(* Logix 5000 AddOnInstructionDefinition export B512_HtoD; software revision 30.00 *)

ADD_ON_INSTRUCTION D_SHR   (* revision 1.0, vendor Ken Fischer, NSWCPD, C512 *)
// DINT bit shift right of the 32-bit argument Inp_A by Inp_B bits with paddding by zeros on the right
// Revision note:
// Rev1.0: TBD - Initial Release
VAR_IN_OUT
   Inp_A : DINT; {required}   // 64-bit Integer to be right circular rotated
END_VAR
VAR_INPUT
   Inp_B : INT; {required}   // Number of bits to shift
END_VAR
VAR_IN_OUT
   Out : DINT; {required}   // Result
END_VAR
VAR
   BSR_Cntrl : CONTROL := (LEN := 32);
   ONS : BOOL;
   Source_Bit : BOOL;
   Wrk_InpA : DINT[2];
END_VAR

ROUTINE Logic   (* ladder *)
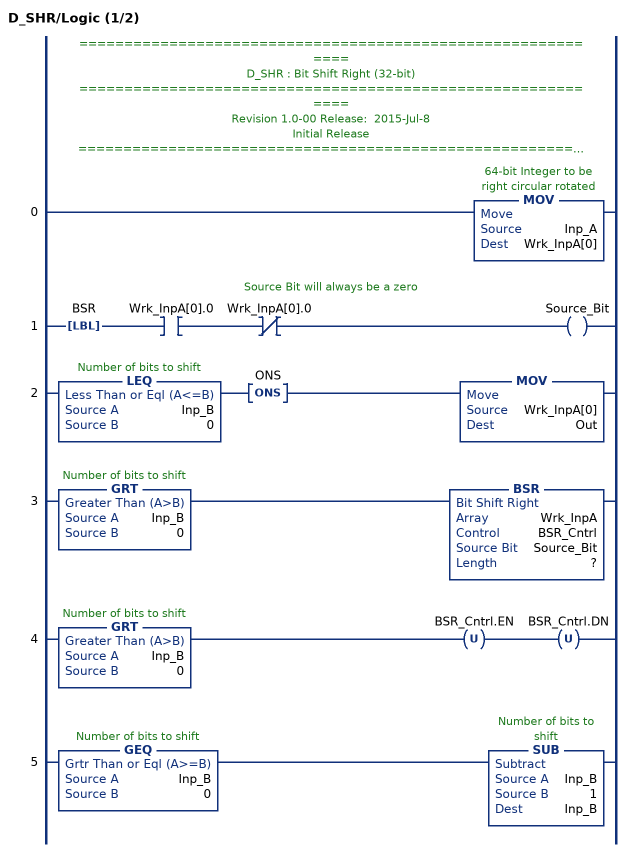
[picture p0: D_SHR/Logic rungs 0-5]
   // ============================================================
   // D_SHR : Bit Shift Right (32-bit)
   // ============================================================
   // Revision 1.0-00 Release:  2015-Jul-8
   // Initial Release
   // ============================================================
   // Performs a right bit shift of the 32-bit argument Inp_A by the
   // number of bits defined in the 16-bit argument Inp_B, with padding by zeros.
   0: MOV(Inp_A,Wrk_InpA[0]);
   // Source Bit will always be a zero
   1: LBL(BSR)XIC(Wrk_InpA[0].0)XIO(Wrk_InpA[0].0)OTE(Source_Bit);
   2: LEQ(Inp_B,0)ONS(ONS)MOV(Wrk_InpA[0],Out);
   3: GRT(Inp_B,0)BSR(Wrk_InpA,BSR_Cntrl,Source_Bit,?);
   4: GRT(Inp_B,0)OTU(BSR_Cntrl.EN)OTU(BSR_Cntrl.DN);
   5: GEQ(Inp_B,0)SUB(Inp_B,1,Inp_B);
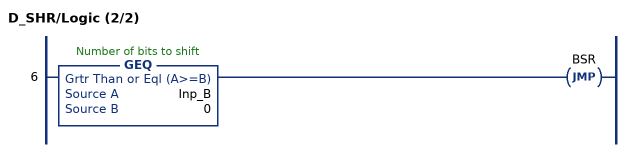
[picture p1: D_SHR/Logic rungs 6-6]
   6: GEQ(Inp_B,0)JMP(BSR);
END_ROUTINE
END_ADD_ON_INSTRUCTION

ADD_ON_INSTRUCTION D_SHL   (* revision 1.0, vendor Ken Fischer, NSWCPD, C512 *)
// DINT bit shift left of the 32-bit argument Inp_A by Inp_B bits with paddding by zeros on the right
// Revision note:
// Rev1.0: TBD - Initial Release
VAR_IN_OUT
   Inp_A : DINT; {required}   // 64-bit Integer to be right circular rotated
END_VAR
VAR_INPUT
   Inp_B : INT; {required}   // Number of bits to shift
END_VAR
VAR_IN_OUT
   Out : DINT; {required}   // Result
END_VAR
VAR
   Wrk_InpA : DINT[2];
   Source_Bit : BOOL;
   ONS : BOOL;
   BSL_Cntrl : CONTROL := (LEN := 32);
END_VAR

ROUTINE Logic   (* ladder *)
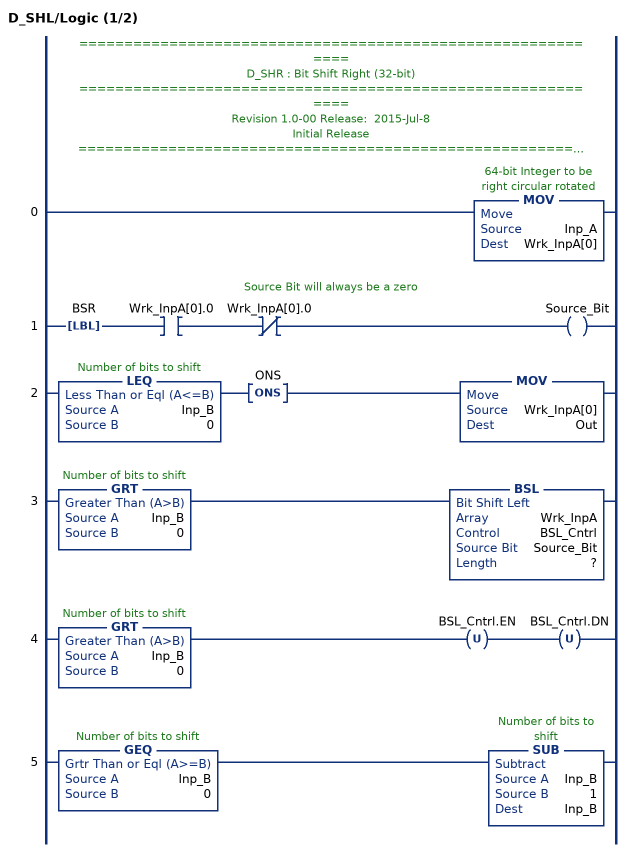
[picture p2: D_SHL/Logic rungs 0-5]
   // ============================================================
   // D_SHR : Bit Shift Right (32-bit)
   // ============================================================
   // Revision 1.0-00 Release:  2015-Jul-8
   // Initial Release
   // ============================================================
   // Performs a left bit shift of the 32-bit argument Inp_A by the
   // number of bits defined in the 16-bit argument Inp_B, with padding by zeros.
   0: MOV(Inp_A,Wrk_InpA[0]);
   // Source Bit will always be a zero
   1: LBL(BSR)XIC(Wrk_InpA[0].0)XIO(Wrk_InpA[0].0)OTE(Source_Bit);
   2: LEQ(Inp_B,0)ONS(ONS)MOV(Wrk_InpA[0],Out);
   3: GRT(Inp_B,0)BSL(Wrk_InpA,BSL_Cntrl,Source_Bit,?);
   4: GRT(Inp_B,0)OTU(BSL_Cntrl.EN)OTU(BSL_Cntrl.DN);
   5: GEQ(Inp_B,0)SUB(Inp_B,1,Inp_B);
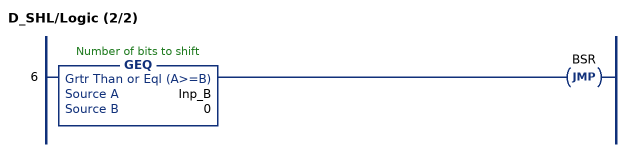
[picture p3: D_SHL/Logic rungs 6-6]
   6: GEQ(Inp_B,0)JMP(BSR);
END_ROUTINE
END_ADD_ON_INSTRUCTION

ADD_ON_INSTRUCTION B512_HtoD   (* revision 1.0 20170916, vendor Kenneth A. Fischer *)
// Takes a 512-bit hash value stored as 8 64-bit pieces and converts it to a 512-bit value stored as 42 12-bit pieces and 1 8-bit piece as the MSB
// Revision note:
// Rev1.0: 20170916 - Initial Release
VAR_IN_OUT
   Inp_H : LINT[8]; {required}
   Out_D : DINT[43]; {required}
END_VAR
VAR
   i : INT := 41;
   j : INT := 62;
   Wrk_InpL : DINT[16];
   D_SHR : D_SHR;
   TEMP1 : DINT;
   D_SHL : D_SHL;
   TEMP2 : DINT;
   EE : DINT[64];
END_VAR

ROUTINE Logic   (* ladder *)
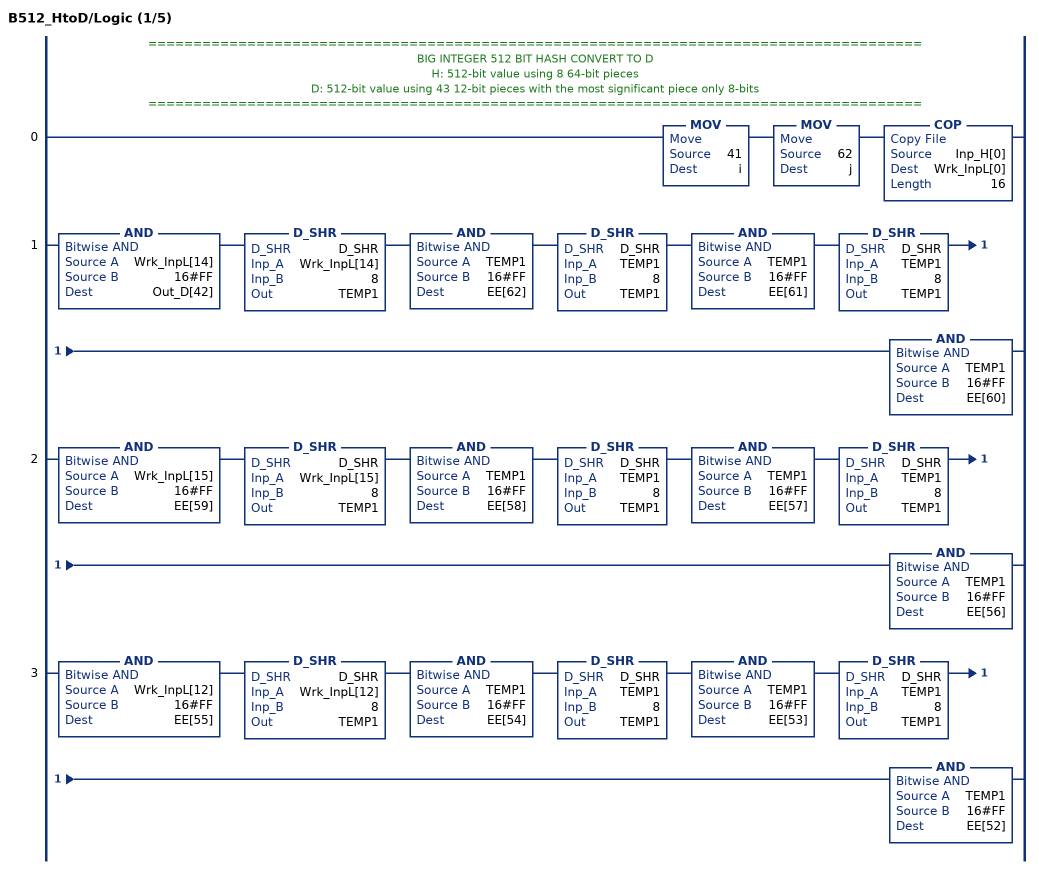
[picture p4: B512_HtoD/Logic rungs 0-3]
   // ======================================================================================
   // BIG INTEGER 512 BIT HASH CONVERT TO D
   // H: 512-bit value using 8 64-bit pieces
   // D: 512-bit value using 43 12-bit pieces with the most significant piece only 8-bits
   // ======================================================================================
   0: MOV(41,i)MOV(62,j)COP(Inp_H[0],Wrk_InpL[0],16);
   1: AND(Wrk_InpL[14],16#FF,Out_D[42])D_SHR(D_SHR,Wrk_InpL[14],8,TEMP1)AND(TEMP1,16#FF,EE[62])D_SHR(D_SHR,TEMP1,8,TEMP1)AND(TEMP1,16#FF,EE[61])D_SHR(D_SHR,TEMP1,8,TEMP1)AND(TEMP1,16#FF,EE[60]);
   2: AND(Wrk_InpL[15],16#FF,EE[59])D_SHR(D_SHR,Wrk_InpL[15],8,TEMP1)AND(TEMP1,16#FF,EE[58])D_SHR(D_SHR,TEMP1,8,TEMP1)AND(TEMP1,16#FF,EE[57])D_SHR(D_SHR,TEMP1,8,TEMP1)AND(TEMP1,16#FF,EE[56]);
   3: AND(Wrk_InpL[12],16#FF,EE[55])D_SHR(D_SHR,Wrk_InpL[12],8,TEMP1)AND(TEMP1,16#FF,EE[54])D_SHR(D_SHR,TEMP1,8,TEMP1)AND(TEMP1,16#FF,EE[53])D_SHR(D_SHR,TEMP1,8,TEMP1)AND(TEMP1,16#FF,EE[52]);
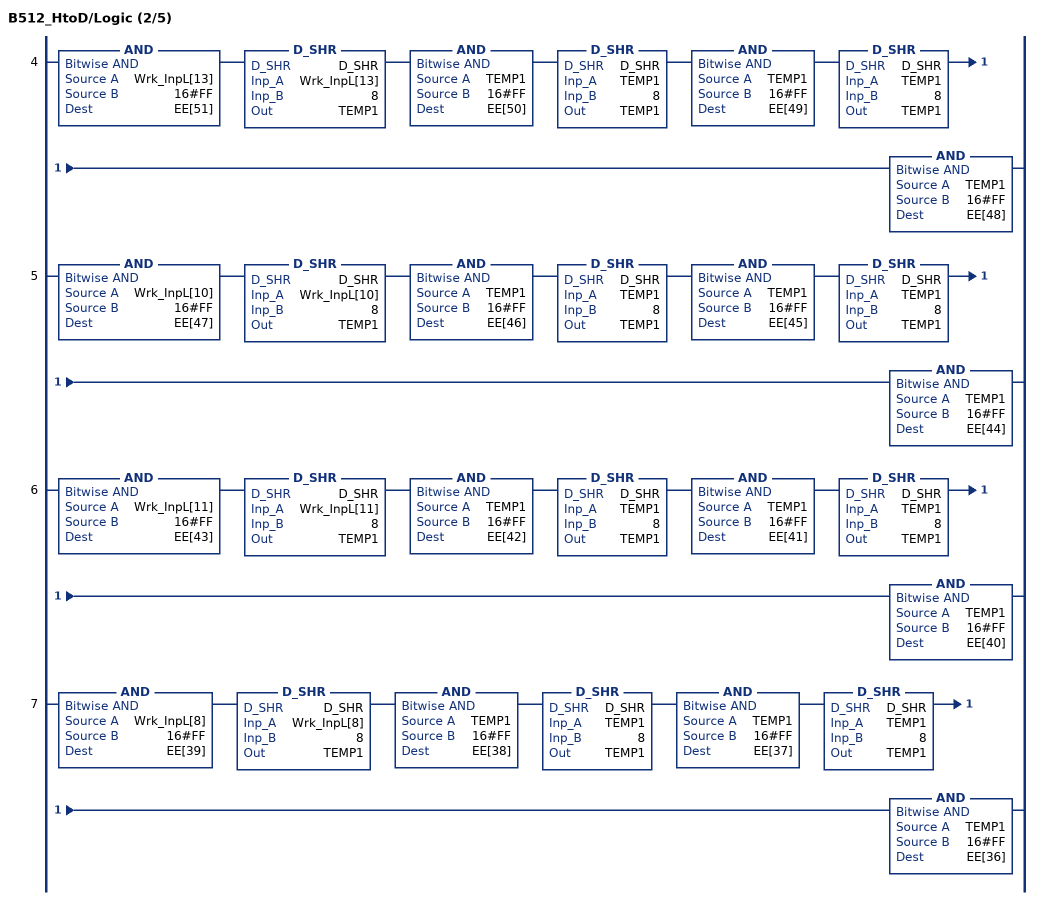
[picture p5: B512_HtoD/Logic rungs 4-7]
   4: AND(Wrk_InpL[13],16#FF,EE[51])D_SHR(D_SHR,Wrk_InpL[13],8,TEMP1)AND(TEMP1,16#FF,EE[50])D_SHR(D_SHR,TEMP1,8,TEMP1)AND(TEMP1,16#FF,EE[49])D_SHR(D_SHR,TEMP1,8,TEMP1)AND(TEMP1,16#FF,EE[48]);
   5: AND(Wrk_InpL[10],16#FF,EE[47])D_SHR(D_SHR,Wrk_InpL[10],8,TEMP1)AND(TEMP1,16#FF,EE[46])D_SHR(D_SHR,TEMP1,8,TEMP1)AND(TEMP1,16#FF,EE[45])D_SHR(D_SHR,TEMP1,8,TEMP1)AND(TEMP1,16#FF,EE[44]);
   6: AND(Wrk_InpL[11],16#FF,EE[43])D_SHR(D_SHR,Wrk_InpL[11],8,TEMP1)AND(TEMP1,16#FF,EE[42])D_SHR(D_SHR,TEMP1,8,TEMP1)AND(TEMP1,16#FF,EE[41])D_SHR(D_SHR,TEMP1,8,TEMP1)AND(TEMP1,16#FF,EE[40]);
   7: AND(Wrk_InpL[8],16#FF,EE[39])D_SHR(D_SHR,Wrk_InpL[8],8,TEMP1)AND(TEMP1,16#FF,EE[38])D_SHR(D_SHR,TEMP1,8,TEMP1)AND(TEMP1,16#FF,EE[37])D_SHR(D_SHR,TEMP1,8,TEMP1)AND(TEMP1,16#FF,EE[36]);
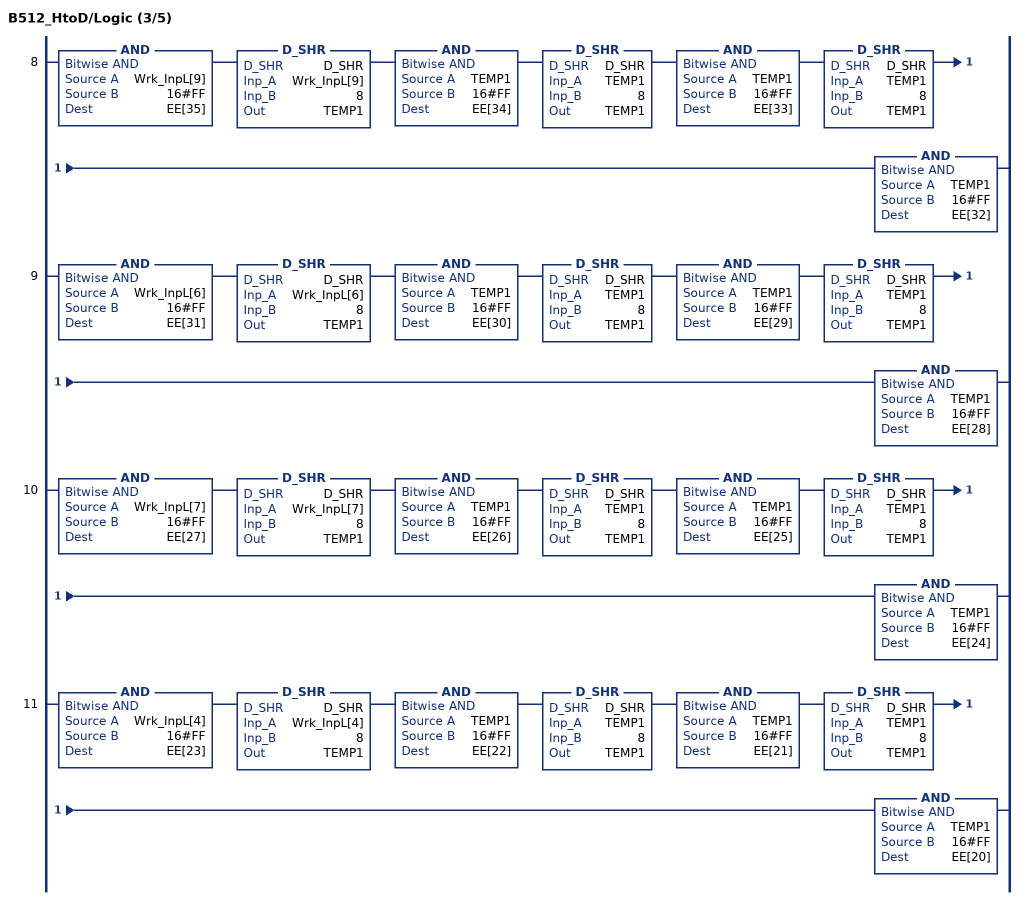
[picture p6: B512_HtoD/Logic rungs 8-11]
   8: AND(Wrk_InpL[9],16#FF,EE[35])D_SHR(D_SHR,Wrk_InpL[9],8,TEMP1)AND(TEMP1,16#FF,EE[34])D_SHR(D_SHR,TEMP1,8,TEMP1)AND(TEMP1,16#FF,EE[33])D_SHR(D_SHR,TEMP1,8,TEMP1)AND(TEMP1,16#FF,EE[32]);
   9: AND(Wrk_InpL[6],16#FF,EE[31])D_SHR(D_SHR,Wrk_InpL[6],8,TEMP1)AND(TEMP1,16#FF,EE[30])D_SHR(D_SHR,TEMP1,8,TEMP1)AND(TEMP1,16#FF,EE[29])D_SHR(D_SHR,TEMP1,8,TEMP1)AND(TEMP1,16#FF,EE[28]);
   10: AND(Wrk_InpL[7],16#FF,EE[27])D_SHR(D_SHR,Wrk_InpL[7],8,TEMP1)AND(TEMP1,16#FF,EE[26])D_SHR(D_SHR,TEMP1,8,TEMP1)AND(TEMP1,16#FF,EE[25])D_SHR(D_SHR,TEMP1,8,TEMP1)AND(TEMP1,16#FF,EE[24]);
   11: AND(Wrk_InpL[4],16#FF,EE[23])D_SHR(D_SHR,Wrk_InpL[4],8,TEMP1)AND(TEMP1,16#FF,EE[22])D_SHR(D_SHR,TEMP1,8,TEMP1)AND(TEMP1,16#FF,EE[21])D_SHR(D_SHR,TEMP1,8,TEMP1)AND(TEMP1,16#FF,EE[20]);
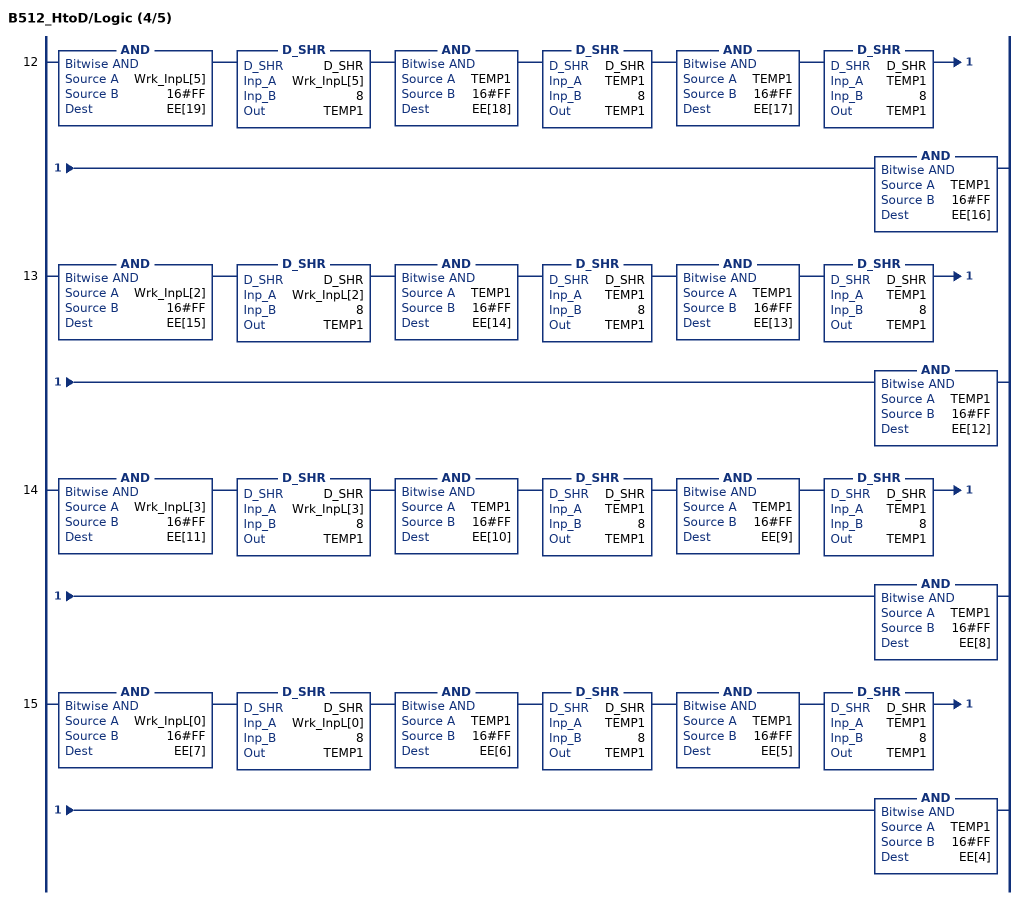
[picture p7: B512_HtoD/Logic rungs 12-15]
   12: AND(Wrk_InpL[5],16#FF,EE[19])D_SHR(D_SHR,Wrk_InpL[5],8,TEMP1)AND(TEMP1,16#FF,EE[18])D_SHR(D_SHR,TEMP1,8,TEMP1)AND(TEMP1,16#FF,EE[17])D_SHR(D_SHR,TEMP1,8,TEMP1)AND(TEMP1,16#FF,EE[16]);
   13: AND(Wrk_InpL[2],16#FF,EE[15])D_SHR(D_SHR,Wrk_InpL[2],8,TEMP1)AND(TEMP1,16#FF,EE[14])D_SHR(D_SHR,TEMP1,8,TEMP1)AND(TEMP1,16#FF,EE[13])D_SHR(D_SHR,TEMP1,8,TEMP1)AND(TEMP1,16#FF,EE[12]);
   14: AND(Wrk_InpL[3],16#FF,EE[11])D_SHR(D_SHR,Wrk_InpL[3],8,TEMP1)AND(TEMP1,16#FF,EE[10])D_SHR(D_SHR,TEMP1,8,TEMP1)AND(TEMP1,16#FF,EE[9])D_SHR(D_SHR,TEMP1,8,TEMP1)AND(TEMP1,16#FF,EE[8]);
   15: AND(Wrk_InpL[0],16#FF,EE[7])D_SHR(D_SHR,Wrk_InpL[0],8,TEMP1)AND(TEMP1,16#FF,EE[6])D_SHR(D_SHR,TEMP1,8,TEMP1)AND(TEMP1,16#FF,EE[5])D_SHR(D_SHR,TEMP1,8,TEMP1)AND(TEMP1,16#FF,EE[4]);
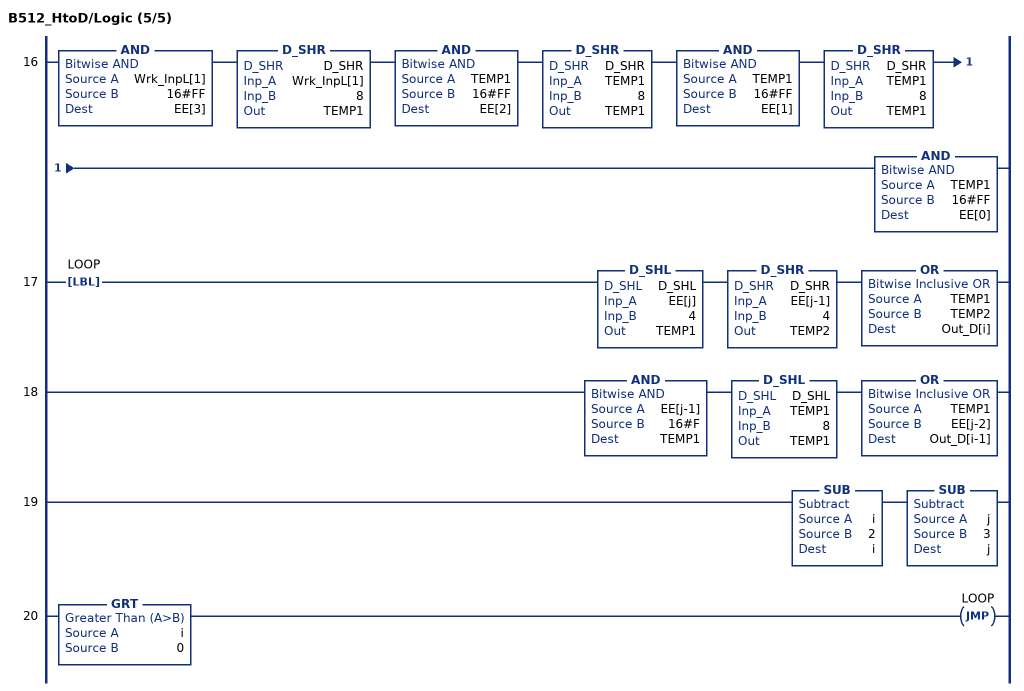
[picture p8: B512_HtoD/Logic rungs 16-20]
   16: AND(Wrk_InpL[1],16#FF,EE[3])D_SHR(D_SHR,Wrk_InpL[1],8,TEMP1)AND(TEMP1,16#FF,EE[2])D_SHR(D_SHR,TEMP1,8,TEMP1)AND(TEMP1,16#FF,EE[1])D_SHR(D_SHR,TEMP1,8,TEMP1)AND(TEMP1,16#FF,EE[0]);
   17: LBL(LOOP)D_SHL(D_SHL,EE[j],4,TEMP1)D_SHR(D_SHR,EE[j-1],4,TEMP2)OR(TEMP1,TEMP2,Out_D[i]);
   18: AND(EE[j-1],16#F,TEMP1)D_SHL(D_SHL,TEMP1,8,TEMP1)OR(TEMP1,EE[j-2],Out_D[i-1]);
   19: SUB(i,2,i)SUB(j,3,j);
   20: GRT(i,0)JMP(LOOP);
END_ROUTINE
END_ADD_ON_INSTRUCTION
